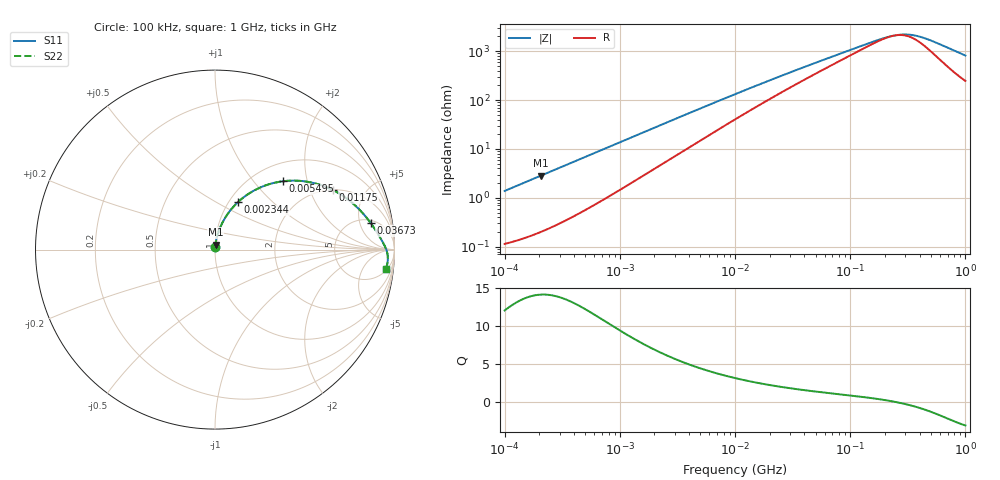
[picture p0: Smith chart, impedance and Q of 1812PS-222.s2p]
# MHz S MA R 50
!Freq  MagS11  AngS11  MagS21  AngS21  MagS12  AngS12  MagS22  AngS22
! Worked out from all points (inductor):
!   801 points, 100 kHz to 1 GHz, reference 50 ohm
!   read as one part in series: L = 2.2 uH near 104.7 kHz
!   highest Q = 14.2 at 206.5 kHz (marker M1), where L = 2.2 uH
!   self-resonance near 240 MHz
!   S11 on the Smith chart (normalised r, x): 100 kHz: 1.00, +0.03; 2.344 MHz: 1.10, +0.63; 5.495 MHz: 1.34, +1.44; 11.75 MHz: 2.01, +2.91; 36.73 MHz: 5.68, +7.47; 1 GHz: 6, -16
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0.1  0.01384 84.5  0.9988 -0.8  0.9988 -0.8  0.01384 84.5
0.206538  0.02849 84.3  0.9976 -1.6  0.9976 -1.6  0.02849 84.3
0.4677351  0.06409 81.8  0.9928 -3.7  0.9928 -3.7  0.06409 81.8
1.148154  0.1533 74.8  0.9712 -8.8  0.9712 -8.8  0.1533 74.8
1.603245  0.2092 70.6  0.9511 -12.0  0.9511 -12.0  0.2092 70.6
2.162719  0.2728 65.8  0.9222 -15.7  0.9222 -15.7  0.2728 65.8
2.344229  0.2922 64.3  0.9122 -16.8  0.9122 -16.8  0.2922 64.3
3.507519  0.402 56.0  0.8435 -23.3  0.8435 -23.3  0.402 56.0
5.495409  0.5382 45.1  0.7275 -31.6  0.7275 -31.6  0.5382 45.1
7.328245  0.6219 37.8  0.6357 -36.9  0.6357 -36.9  0.6219 37.8
10  0.7007 30.4  0.5311 -41.9  0.5311 -41.9  0.7007 30.4
11.74898  0.7354 26.8  0.4781 -44.0  0.4781 -44.0  0.7354 26.8
19.95262  0.8211 17.2  0.3246 -48.4  0.3246 -48.4  0.8211 17.2
36.72823  0.8796 9.7  0.1996 -48.2  0.1996 -48.2  0.8796 9.7
46.77351  0.8955 7.7  0.164 -46.7  0.164 -46.7  0.8955 7.7
154.8817  0.944 1.5  0.06134 -23.3  0.06134 -23.3  0.944 1.5
216.2719  0.9521 0.3  0.04826 -6.8  0.04826 -6.8  0.9521 0.3
288.4032  0.9577 -0.6  0.04361 13.5  0.04361 13.5  0.9577 -0.6
331.1311  0.9598 -1.1  0.04424 24.2  0.04424 24.2  0.9598 -1.1
380.1894  0.9616 -1.6  0.04692 34.4  0.04692 34.4  0.9616 -1.6
501.1872  0.964 -2.7  0.0582 50.5  0.0582 50.5  0.964 -2.7
1000  0.9581 -6.4  0.1175 65.9  0.1175 65.9  0.9581 -6.4
